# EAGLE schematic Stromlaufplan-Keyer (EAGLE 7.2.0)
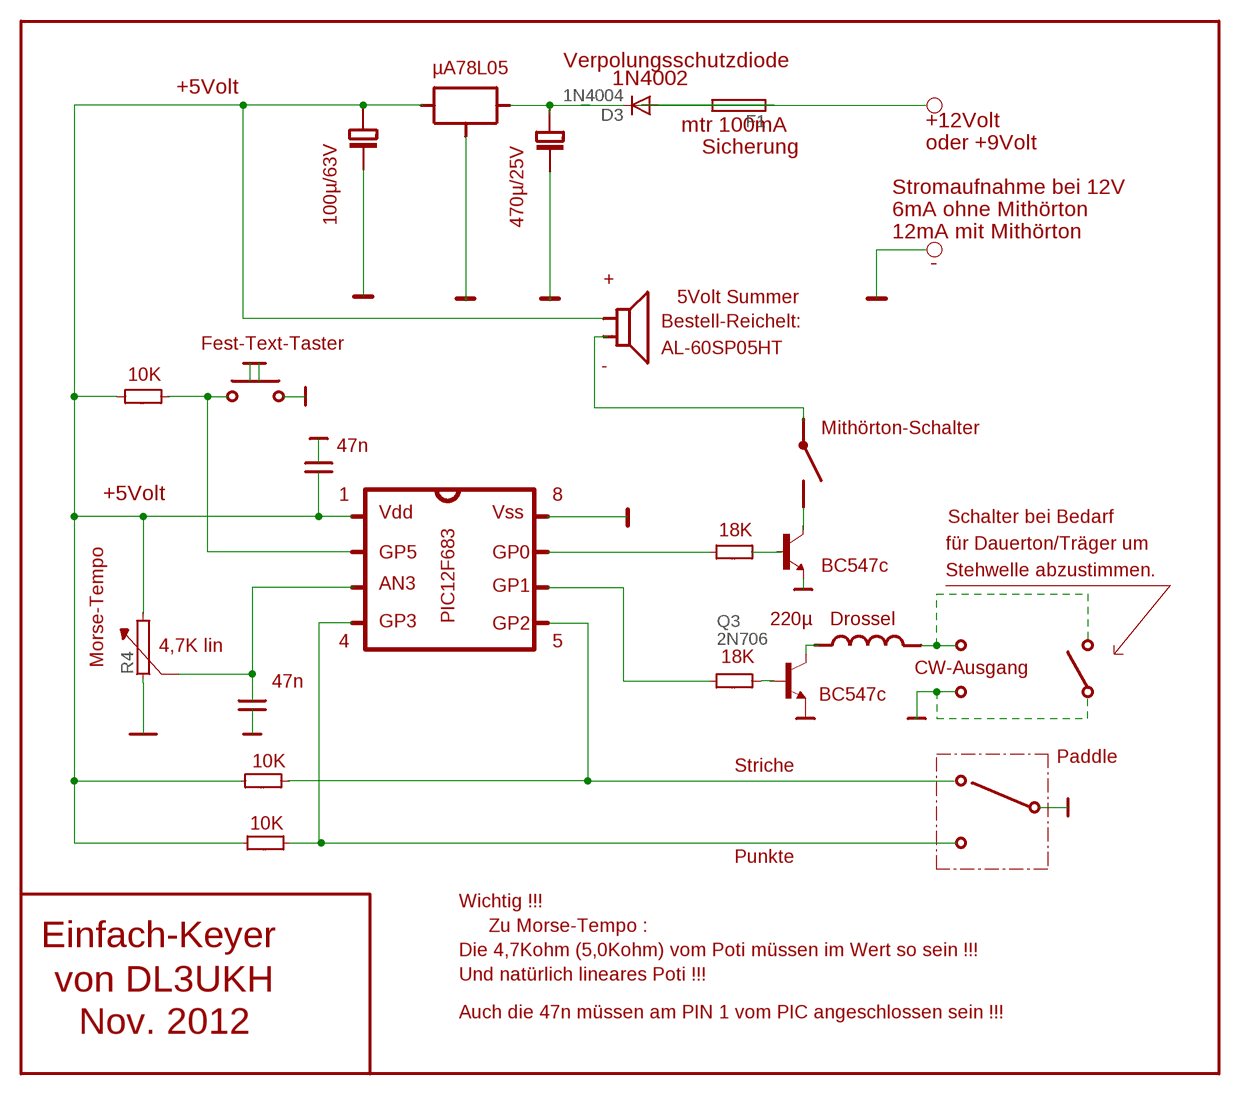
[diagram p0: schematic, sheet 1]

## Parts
D3  1N4004  [DO41-10]
F1  19559  [19559]
Q3  2N706  [TO18]
R4  RHS10  [HS10]

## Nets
N$8: D3.C
N$20: R4.2
N$34: Q3.2(B)
N$37: Q3.3(C)
N$47: D3.A F1.1 F1.2
N$72: R4.1
Unconnected: Q3.1(E)

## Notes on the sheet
- Verpolungsschutzdiode
- +5Volt | µA78L05
- 1N4002
- mtr 100mA | +12Volt
- Sicherung
- oder +9Volt
- Stromaufnahme bei 12V
- 6mA ohne Mithörton
- 100µ/63V | 470µ/25V
- 12mA mit Mithörton
- -
- + | 5Volt Summer
- Bestell-Reichelt:
- Fest-Text-Taster | AL-60SP05HT
- -
- 10K
- Mithörton-Schalter
- 47n
- +5Volt
- 1 | 8
- Vdd | Vss | Schalter bei Bedarf
- 18K
- für Dauerton/Träger um
- GP5 | GP0
- BC547c | Stehwelle abzustimmen.
- AN3 | GP1
- GP3 | PIC12F683 | 220µ | Drossel
- GP2
- 4,7K lin | 4 | 5
- Morse-Tempo | 18K
- 47n | CW-Ausgang
- BC547c
- 10K | Paddle
- Striche
- 10K
- Punkte
- Wichtig !!!
- Zu Morse-Tempo :
- Einfach-Keyer
- Die 4,7Kohm (5,0Kohm) vom Poti müssen im Wert so sein !!!
- Und natürlich lineares Poti !!!
- von DL3UKH
- Auch die 47n müssen am PIN 1 vom PIC angeschlossen sein !!!
- Nov. 2012

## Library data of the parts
D3 = diode:1N4004: DIODE
F1 = fuse:19559: FUSE HOLDER
Q3 = transistor-npn:2N706: NPN Transistor
R4 = resistor-power:R: Power Resitor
